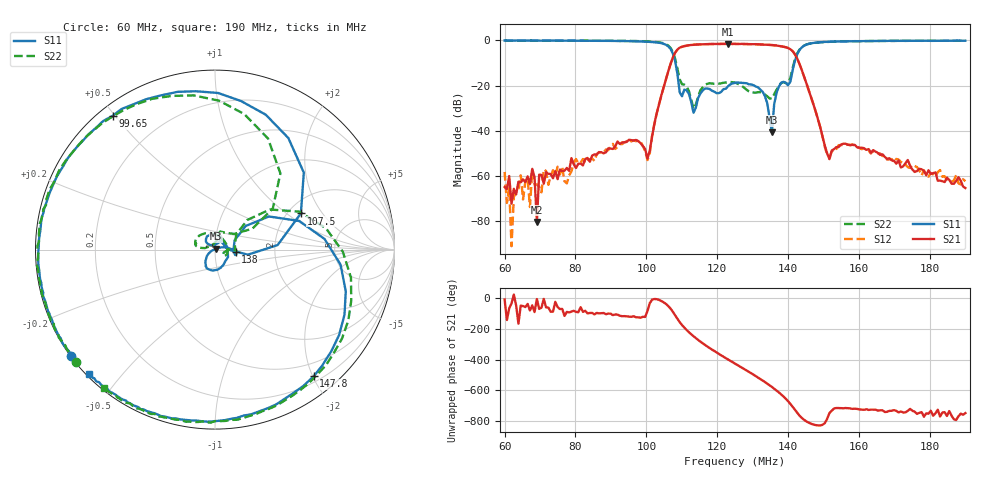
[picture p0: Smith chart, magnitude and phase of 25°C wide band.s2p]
!Agilent Technologies,E8362C,SG49020144,A.09.33.09
!Agilent E8362C: A.09.33.09
!Date: Friday, October 10, 2025 09:27:13
!Correction: S11(Full 2 Port(1,2))
!S21(Full 2 Port(1,2))
!S12(Full 2 Port(1,2))
!S22(Full 2 Port(1,2))
!S2P File: Measurements: S11, S21, S12, S22:
# Hz S  dB  R 50
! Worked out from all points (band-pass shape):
!   201 points, 60 MHz to 190 MHz, reference 50 ohm
!   highest |S21| = -1.50 dB at 123 MHz (marker M1); lowest = -80.3 dB at 69.1 MHz (marker M2)
!   |S21| within 3 dB of the highest: 108.5 MHz to 141.1 MHz (32.55 MHz wide, 26.1 % of centre)
!   lowest |S11| = -40.7 dB at 135.4 MHz (marker M3), VSWR 1.02, Z = 50.7 + j0.557 ohm
!   |S11| at or under -10 dB: 108.2 MHz to 141.8 MHz (33.55 MHz wide, 26.8 % of centre)
!   |S22| runs from -30.2 to 0.0 dB; largest |S21 - S12| = 0.0082
!   S11 on the Smith chart (normalised r, x): 60 MHz: 0.00, -0.33; 99.65 MHz: 0.04, +0.49; 107.5 MHz: 2.34, +1.29; 138 MHz: 1.26, -0.04; 147.8 MHz: 0.28, -2.01; 190 MHz: 0.01, -0.41
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6e7  -0.04 -143.6  -64.80 -7.6  -58.15 -16.4  -0.05 -141.0
6.195e7  -0.05 -146.6  -72.16 -33.8  -90.95 -82.1  -0.06 -143.7
6.455e7  -0.08 -150.0  -62.67 -47.2  -59.61 -86.0  -0.08 -147.3
6.715e7  -0.07 -154.1  -63.50 -79.4  -73.67 -26.4  -0.01 -150.6
6.78e7  -0.06 -155.4  -56.77 -45.8  -57.59 -38.2  -0.06 -151.5
6.91e7  -0.09 -156.8  -80.28 -4.9  -63.65 -28.5  -0.02 -153.1
6.975e7  -0.08 -158.2  -59.30 -69.1  -64.71 -10.0  -0.04 -154.3
8.21e7  -0.13 -178.3  -55.24 -88.8  -52.43 -73.8  -0.07 -172.9
9.965e7  -0.55 127.5  -47.99 -121.7  -48.90 -122.2  -0.40 139.0
1.0355e8  -1.03 96.9  -28.37 -10.0  -28.25 -10.4  -0.82 112.6
1.0745e8  -5.69 22.9  -7.59 -87.4  -7.66 -87.4  -5.04 49.4
1.107e8  -21.75 68.7  -2.50 168.7  -2.54 168.3  -19.53 73.8
1.146e8  -25.47 141.7  -1.79 87.9  -1.75 88.0  -24.87 171.8
1.2305e8  -20.25 -61.0  -1.50 -39.9  -1.55 -39.8  -18.46 156.6
1.25e8  -18.75 -91.6  -1.56 -66.6  -1.54 -66.3  -18.59 138.2
1.354e8  -40.66 36.3  -2.03 141.3  -2.05 141.3  -25.77 -18.8
1.38e8  -18.76 -7.0  -2.54 93.0  -2.57 93.2  -18.90 -1.9
1.471e8  -1.11 -47.2  -28.18 -104.5  -28.11 -104.7  -1.14 -40.9
1.4775e8  -0.97 -52.1  -31.34 -108.2  -31.40 -107.8  -0.99 -46.0
1.5165e8  -0.59 -74.9  -52.49 -29.0  -51.52 -32.4  -0.59 -68.4
1.6855e8  -0.17 -115.0  -52.09 -15.5  -52.54 -15.3  -0.14 -108.8
1.9e8  -0.13 -135.4  -65.26 -29.8  -62.24 -17.9  -0.10 -128.6
